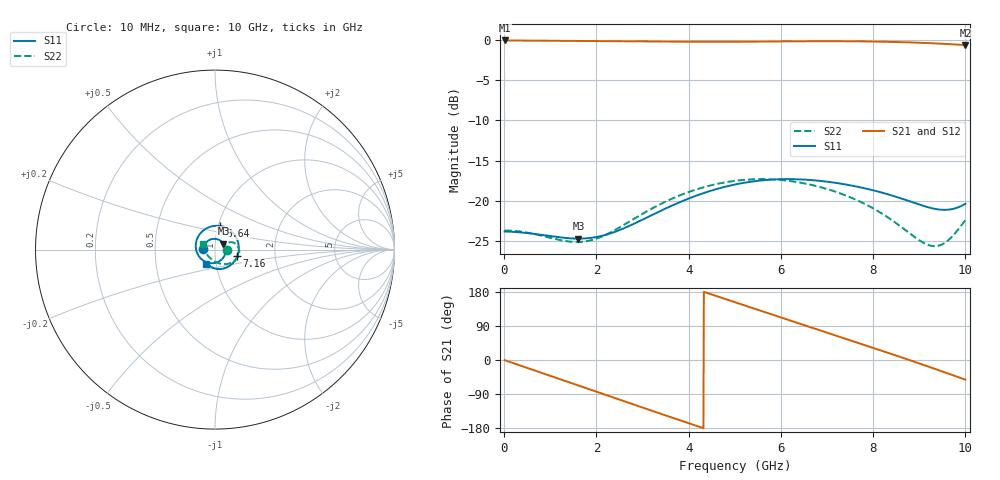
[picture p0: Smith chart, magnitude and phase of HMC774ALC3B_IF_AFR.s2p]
! Analog Devices, Inc.
! 1 Analog Way
! Wilmington, MA 01887
! http://www.analog.com
! Date:  2021-09-17 NN
! Board Name:  EV1HMC774ALC3B Revision A with HMC774ALC3B installed
! File Description:  Automatic Fixture Removal S-Parameters for IF Port connector and board loss de-embedding
! File Generation:  Calibrated Network Analyzer
! Chip Part Number:  HMC774ALC3B
! Chip Description:  MMIC, Double Balanced Mixer
! Chip Frequency:  7 to 34 GHz
! Chip Package:  LCC, 2.9 x 2.9 x 0.8 mm
! IF Port:  HMC774ALC3B removed and end of trace left open
! Note:
!  Analog Devices supplies this data as a sample of measured data at the evaluation board
!  ports for this product.  Your particular data for this product may vary.
!  Analog Devices reserves the right to change this data at anytime.
!  All lines below in this file are as is from the Network Analyzer.
!Agilent Technologies,N5245A,MY52451809,A.10.47.06
!Automatic Fixture Removal (AFR)
!Date: Friday, September 17, 2021 5:44:22 AM
!S2P File: Measurements: S11,S21,S12,S22:
# MHz S  RI  R 50
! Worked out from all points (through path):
!   1000 points, 10 MHz to 10 GHz, reference 50 ohm
!   highest |S21| = -0.02 dB at 10 MHz (marker M1); lowest = -0.6 dB at 10 GHz (marker M2)
!   group delay of S21, straight-line fit = 114 ps
!   lowest |S11| = -24.7 dB at 1.61 GHz (marker M3), VSWR 1.12, Z = 54.8 + j3.72 ohm
!   |S11| at or under -10 dB: start of sweep to end of sweep
!   |S22| runs from -25.7 to -17.3 dB; largest |S21 - S12| = 1.4e-15
!   S11 on the Smith chart (normalised r, x): 10 MHz: 0.88, +0.00; 5.64 GHz: 1.03, +0.27; 7.16 GHz: 1.28, -0.10; 10 GHz: 0.89, -0.15
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10  -0.0642 0.000944  0.9978 -0.0073  0.9978 -0.0073  0.0651 -3.43e-05
760  -0.0259 0.0557  0.8449 -0.5247  0.8449 -0.5247  0.061 -0.000524
1610  0.0471 0.0338  0.3799 -0.9158  0.3799 -0.9158  0.0543 0.0103
1680  0.0509 0.0279  0.3324 -0.9338  0.3324 -0.9338  0.0541 0.0117
2080  0.0589 -0.0112  0.0491 -0.9881  0.0491 -0.9881  0.0554 0.0207
2480  0.0424 -0.0495  -0.2366 -0.9583  -0.2366 -0.9583  0.0607 0.0297
2890  0.00426 -0.0734  -0.5065 -0.8446  -0.5065 -0.8446  0.0701 0.0371
3340  -0.0479 -0.0701  -0.7482 -0.6365  -0.7482 -0.6365  0.0841 0.0412
3770  -0.0894 -0.037  -0.9047 -0.3778  -0.9047 -0.3778  0.0991 0.0397
4180  -0.107 0.0134  -0.974 -0.1001  -0.974 -0.1001  0.1131 0.0331
4590  -0.0961 0.0681  -0.9614 0.1837  -0.9614 0.1837  0.1248 0.0216
5010  -0.0573 0.1124  -0.8664 0.4568  -0.8664 0.4568  0.1328 0.00571
5640  0.0305 0.1307  -0.5896 0.7857  -0.5896 0.7857  0.1343 -0.0226
6160  0.0972 0.0956  -0.2732 0.9468  -0.2732 0.9468  0.125 -0.0455
6670  0.1308 0.0306  0.0736 0.984  0.0736 0.984  0.1079 -0.0637
7160  0.1241 -0.0369  0.3998 0.9024  0.3998 0.9024  0.086 -0.0754
7790  0.0715 -0.0963  0.7461 0.6421  0.7461 0.6421  0.0525 -0.0807
8340  0.0142 -0.1082  0.929 0.3073  0.929 0.3073  0.02 -0.0753
8740  -0.0178 -0.0986  0.9711 0.0303  0.9711 0.0303  -0.00487 -0.064
9140  -0.0361 -0.0845  0.9298 -0.2483  0.9298 -0.2483  -0.0296 -0.0449
9530  -0.0434 -0.0761  0.8104 -0.4974  0.8104 -0.4974  -0.0513 -0.0169
10000  -0.0508 -0.081  0.5757 -0.735  0.5757 -0.735  -0.0692 0.0309
